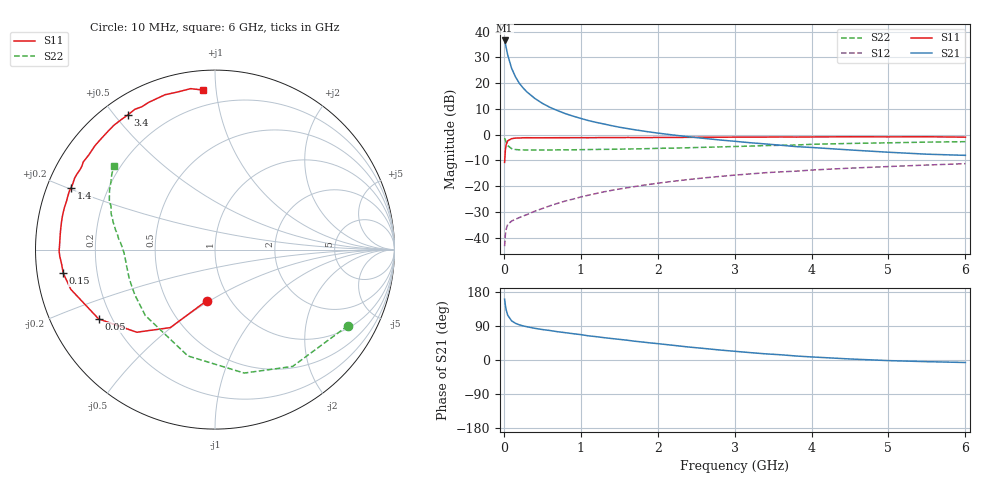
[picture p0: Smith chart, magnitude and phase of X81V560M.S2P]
! SIEMENS Small Signal Semiconductors
! BFP136W
! Si NPN RF Bipolar Junction Transistor in SOT343
! VCE = 1.5 V  IC = 60 mA
! Common Emitter S-Parameters:  September  1994
# GHz  S  MA  R  50
!  f  S11  S21  S12  S22
! GHz  MAG  ANG  MAG  ANG  MAG  ANG  MAG  ANG
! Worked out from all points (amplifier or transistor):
!   40 points, 10 MHz to 6 GHz, reference 50 ohm
!   highest |S21| = 36.6 dB at 10 MHz (marker M1)
!   |S21| within 3 dB of that: start of sweep to 31.97 MHz
!   unconditionally stable (mu >= 1): 549.5 MHz to 2.908 GHz
!   at 200 MHz: K = 0.61, MSG = 26.1 dB, |S12| = -32.3 dB
!   at 1.5 GHz: K = 1.12, MAG = 9.9 dB, |S12| = -21.1 dB
!   at 6 GHz: K = 0.99, MSG = 1.6 dB, |S12| = -11.3 dB
!   S11 on the Smith chart (normalised r, x): 10 MHz: 0.78, -0.48; 50 MHz: 0.15, -0.27; 150 MHz: 0.08, -0.08; 1.4 GHz: 0.07, +0.21; 3.4 GHz: 0.07, +0.54; 6 GHz: 0.11, +0.92
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0.01  0.2888 -99.3  67.35 160.6  0.0068 70.7  0.8531 -29.8
0.02  0.5008 -119.8  58.16 144.3  0.0114 57.6  0.7815 -56.4
0.03  0.6338 -133.4  49.27 132.6  0.0145 48.1  0.7068 -76.7
0.05  0.7546 -149.2  35.31 118.3  0.0179 37.6  0.6115 -104.3
0.1  0.8334 -164.6  19.59 103.6  0.0209 32.0  0.5344 -136.6
0.15  0.8554 -171.1  13.32 96.9  0.0226 34.2  0.5131 -150.3
0.2  0.8586 -174.7  9.997 92.9  0.0244 36.0  0.5058 -157.6
0.25  0.8658 -177.6  8.071 90.0  0.0262 39.3  0.5037 -162.2
0.3  0.8686 -179.4  6.744 87.8  0.0279 42.0  0.5011 -165.4
0.4  0.8658 176.9  5.074 83.7  0.0324 46.4  0.501 -169.5
0.5  0.8665 174.3  4.049 80.4  0.0366 50.1  0.5014 -172.3
0.6  0.8674 172.3  3.377 77.8  0.0414 52.8  0.5026 -174.1
0.7  0.869 169.7  2.914 74.6  0.0462 55.4  0.5043 -175.3
0.9  0.8708 166.1  2.281 69.4  0.0558 57.4  0.5068 -177.8
1.1  0.8703 161.8  1.869 63.8  0.0665 58.5  0.5117 -179.5
1.4  0.8727 156.7  1.491 56.7  0.0824 58.7  0.5181 178.2
2.2  0.879 143.0  0.982 38.8  0.1239 54.4  0.5459 172.1
3.2  0.8929 126.0  0.695 19.5  0.1719 45.4  0.597 163.1
3.4  0.8941 122.8  0.658 16.3  0.1817 43.3  0.6114 161.1
4.5  0.9066 107.9  0.503 2.7  0.2228 33.1  0.6732 150.8
5.5  0.907 98.6  0.416 -4.4  0.2562 25.1  0.7138 143.6
6  0.8914 94.3  0.395 -6.6  0.2724 20.6  0.7283 140.4
